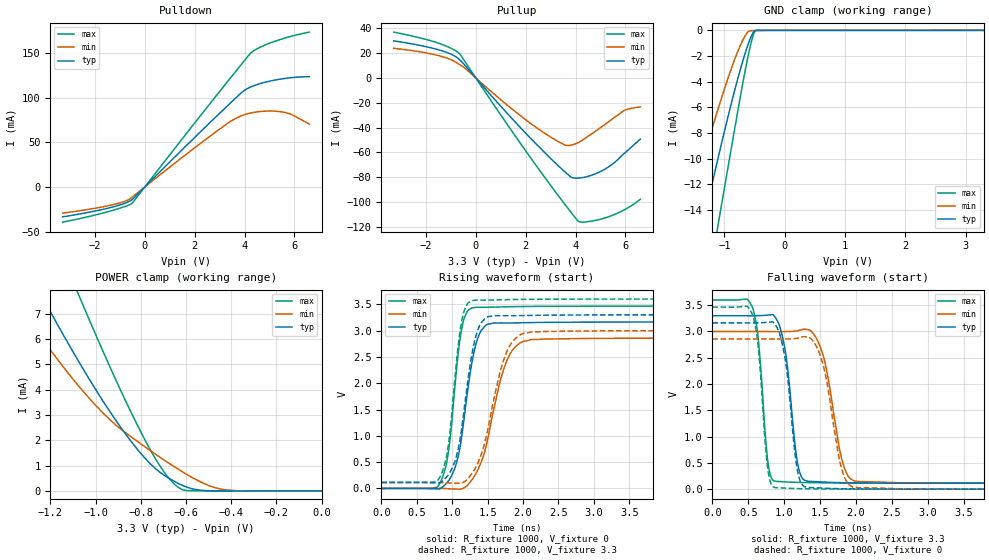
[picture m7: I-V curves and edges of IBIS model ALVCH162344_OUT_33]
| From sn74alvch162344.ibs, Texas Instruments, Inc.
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[Model]   ALVCH162344_OUT_33
Model_type  3-state
Enable   Active-Low
Vref =   0
Rref =   500
Cref =   50p
Vmeas =   1.5
| variable   typ   min   max
C_comp   3.57pF   3.17pF   3.85pF
| C_pullup   1.22pF   0.91pF   1.87pF
| C_pulldown   0.77pF   0.67pF   0.95pF
| C_tri-state   3.57pF   3.17pF   3.85pF
[Temperature Range]   40   100   -40
| Ambient temperature   25   85   -40
[Voltage range]   3.3   3   3.6
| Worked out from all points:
|   slope of the pulldown table from 0 to 0.495 V, typ, clamps not added: 35.7 ohm
|   slope of the pullup table from 0 to 0.495 V, typ, clamps not added: 43.4 ohm
|   GND clamp passes 1 mA (typ) near -0.60 V on its own axis
|   POWER clamp passes 1 mA (typ) near -0.75 V on its own axis
|   rising waveform, R_fixture 1000, V_fixture 0: 20-80 % time 211ps typ, 304ps min, 158ps max; typ from 0 V to 3.16 V
|   falling waveform, R_fixture 1000, V_fixture 3.3: 20-80 % time 148ps typ, 217ps min, 115ps max; typ from 3.3 V to 0.114 V
|   rising waveform, R_fixture 1000, V_fixture 3.3: 20-80 % time 210ps typ, 303ps min, 157ps max; typ from 0.113 V to 3.3 V
|   falling waveform, R_fixture 1000, V_fixture 0: 20-80 % time 147ps typ, 211ps min, 114ps max; typ from 3.16 V to 0 V
[GND Clamp]
| ALVCH162344_OUT_33
|   Voltage   I(typ)   I(min)   I(max)
-3.3V     -59.28mA   -44.88mA   -79.72mA
-1.68V    -22.11mA   -15.5mA    -31.37mA
-1.625V   -20.9mA    -14.56mA   -29.78mA
-1.385V   -15.74mA   -10.55mA   -22.95mA
-1.34V    -14.79mA   -9.816mA   -21.68mA
-1.11V    -10.05mA   -6.197mA   -15.29mA
-790mV    -3.97mA    -1.778mA   -6.606mA
-665mV    -1.915mA   -497.2uA   -3.359mA
-585mV    -803.7uA   -47.18uA   -1.514mA
-515mV    -114.9uA   -19.3uA    -279.6uA
-465mV    -9.965uA   -12.2uA    -8.146uA
3.3V      111.1pA    1.109uA    48.01pA
[POWER Clamp]
| ALVCH162344_OUT_33
|   Voltage   I(typ)   I(min)   I(max)
-3.3V     48.32mA    38.34mA    63.61mA
-1.365V   9.848mA    7.65mA     14.17mA
-1.25V    7.901mA    6.177mA    11.57mA
-1.22V    7.407mA    5.809mA    10.9mA
-1.07V    5.042mA    4.093mA    7.644mA
-925mV    2.98mA     2.72mA     4.675mA
-805mV    1.537mA    1.892mA    2.419mA
-715mV    735uA      1.33mA     985.6uA
-645mV    346.5uA    917uA      221uA
-600mV    161.8uA    669.2uA    18.48uA
-430mV    670.8nA    50.8uA     22.89nA
-48.03fV  111.1pA    335.1pA    59.08pA
[Pulldown]
| ALVCH162344_OUT_33
|   Voltage   I(typ)   I(min)   I(max)
-3.3V     -33.65mA   -29.39mA   -39.57mA
-1.34V    -22.89mA   -20.34mA   -26.72mA
-800mV    -18.34mA   -16.09mA   -22.02mA
-525mV    -14.57mA   -11.78mA   -18.54mA
2.65V     73.08mA    57.53mA    94.6mA
3.45V     94.44mA    73.68mA    122.6mA
3.9V      106.1mA    79.97mA    138.3mA
4.22V     111.6mA    82.67mA    149.2mA
4.375V    113.4mA    83.51mA    152.7mA
5.43V     120.7mA    84.32mA    165.1mA
5.875V    122.4mA    81.21mA    168.8mA
6.6V      123.5mA    70.36mA    173.5mA
[Pullup]
| ALVCH162344_OUT_33
|   Voltage   I(typ)   I(min)   I(max)
-3.3V     30mA       24.03mA    37.09mA
-1.495V   22.81mA    18.08mA    28.11mA
-980mV    19.12mA    14.67mA    23.89mA
-665mV    15.03mA    11.05mA    19.72mA
2.35V     -51.83mA   -38.82mA   -68.65mA
3.475V    -73.88mA   -53.03mA   -99.32mA
3.84V     -80.11mA   -53.99mA   -108.9mA
4.155V    -80.61mA   -51.49mA   -115.9mA
4.765V    -77.48mA   -43.33mA   -114.9mA
5.375V    -70.94mA   -34.56mA   -111.5mA
5.925V    -61.27mA   -26.48mA   -106.6mA
6.6V      -49.2mA    -23.27mA   -97.77mA
[Ramp]
| ALVCH162344_OUT_33
| variable   typ   min   max
dV/dt_r   1.90/2.18E-10   1.72/3.16E-10   2.08/1.61E-10
dV/dt_f   1.93/1.54E-10   1.76/2.28E-10   2.10/1.20E-10
R_load = 1000
[Rising Waveform]
| ALVCH162344_OUT_33
R_fixture =   1000
C_fixture =   0
L_fixture =   0
V_fixture =   0
V_fixture_min = 0
V_fixture_max = 0
|   Time   V(typ)   V(min)   V(max)
0s        -3.555uV   -3.49uV    -2.514uV
830ps     -1.272mV   752.9uV    107.2mV
950ps     150.2mV    -5.193mV   726.2mV
1.055ns   459.7mV    -12.25mV   2.175V
1.14ns    1.039V     -5.169mV   3.072V
1.335ns   2.741V     281.4mV    3.442V
1.485ns   3.11V      840.6mV    3.444V
1.78ns    3.145V     2.458V     3.454V
2.145ns   3.154V     2.833V     3.461V
25ns      3.163V     2.858V     3.465V
[Falling Waveform]
| ALVCH162344_OUT_33
R_fixture =   1000
C_fixture =   0
L_fixture =   0
V_fixture =   3.3
V_fixture_min = 3
V_fixture_max = 3.6
|   Time   V(typ)   V(min)   V(max)
0s        3.3V       3V         3.6V
565ps     3.298V     3V         3.438V
645ps     3.301V     3V         2.776V
775ps     3.312V     2.999V     501.6mV
880ps     3.262V     2.998V     149.4mV
1.02ns    2.599V     2.999V     138.3mV
1.19ns    470.5mV    3.015V     128.5mV
1.33ns    149.9mV    3.037V     124.5mV
1.995ns   118.8mV    150.2mV    118.2mV
25ns      113.5mV    111.5mV    117.3mV
[Rising Waveform]
| ALVCH162344_OUT_33
R_fixture =   1000
C_fixture =   0
L_fixture =   0
V_fixture =   3.3
V_fixture_min = 3
V_fixture_max = 3.6
|   Time   V(typ)   V(min)   V(max)
0s        113.5mV    111.5mV    117.3mV
830ps     112.5mV    111.6mV    226mV
945ps     258mV      106.3mV    811.2mV
1.065ns   640mV      99.23mV    2.471V
1.16ns    1.405V     119.4mV    3.333V
1.29ns    2.635V     306.2mV    3.573V
1.46ns    3.225V     869.8mV    3.58V
1.775ns   3.282V     2.612V     3.589V
2.135ns   3.29V      2.978V     3.596V
25ns      3.3V       3V         3.6V
[Falling Waveform]
| ALVCH162344_OUT_33
R_fixture =   1000
C_fixture =   0
L_fixture =   0
V_fixture =   0
V_fixture_min = 0
V_fixture_max = 0
|   Time   V(typ)   V(min)   V(max)
0s        3.163V     2.858V     3.465V
565ps     3.162V     2.858V     3.299V
640ps     3.164V     2.858V     2.693V
770ps     3.175V     2.857V     407.7mV
875ps     3.132V     2.856V     29.22mV
1.02ns    2.43V      2.858V     19.45mV
1.19ns    318.9mV    2.874V     10.33mV
1.325ns   31.91mV    2.895V     6.754mV
1.98ns    4.822mV    32.68mV    796.3uV
25ns      294.3nV    359.7nV    274.8nV
